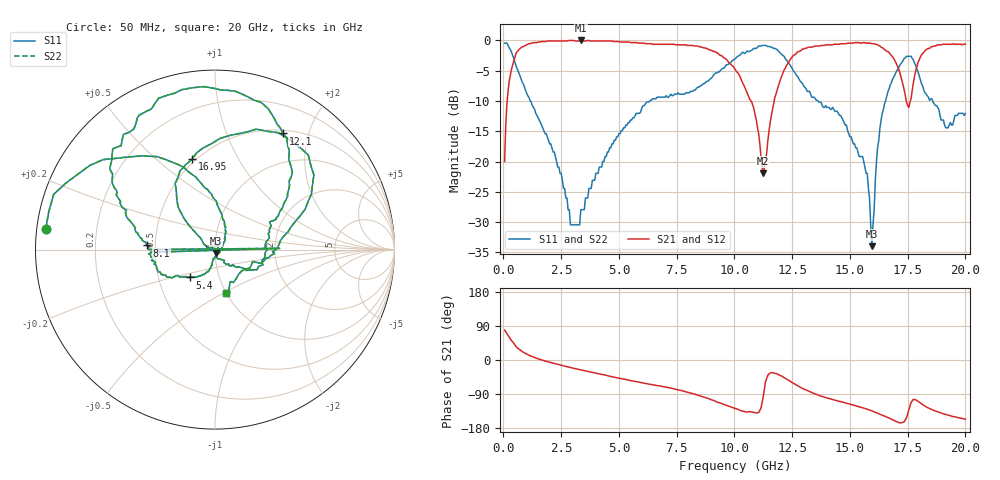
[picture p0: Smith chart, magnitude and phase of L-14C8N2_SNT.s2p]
#	mhz	s	ma	r	50
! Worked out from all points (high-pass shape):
!   400 points, 50 MHz to 20 GHz, reference 50 ohm
!   highest |S21| = 0.00 dB at 3.35 GHz (marker M1); lowest = -21.9 dB at 11.25 GHz (marker M2)
!   |S21| within 3 dB of the highest: 478.4 MHz to 9.61 GHz (9.132 GHz wide, 181 % of centre); 12.44 GHz to 16.9 GHz (4.458 GHz wide, 30.4 % of centre)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
!   lowest |S11| = -34.0 dB at 15.95 GHz (marker M3), VSWR 1.04, Z = 50.7 - j1.9 ohm
!   |S11| at or under -10 dB: 1.169 GHz to 6.331 GHz (5.163 GHz wide, 138 % of centre); 13.62 GHz to 16.54 GHz (2.922 GHz wide, 19.4 % of centre); 18.58 GHz to end of sweep
!   |S22| runs from -34.0 to -0.4 dB; largest |S21 - S12| = 0
!   S11 on the Smith chart (normalised r, x): 50 MHz: 0.03, +0.06; 5.4 GHz: 0.72, -0.23; 8.1 GHz: 0.45, +0.02; 12.1 GHz: 0.54, +1.61; 16.95 GHz: 0.48, +0.66; 20 GHz: 1.00, -0.52
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50  0.95 173.2  0.1 79.0  0.1 79.0  0.95 173.2
550  0.61 121.9  0.79 34.9  0.79 34.9  0.61 121.9
2900  0.03 6.3  1 -19.9  1 -19.9  0.03 6.3
3350  0.04 -81.1  1 -26.3  1 -26.3  0.04 -81.1
3400  0.04 -84.2  1 -26.9  1 -26.9  0.04 -84.2
5400  0.21 -132.3  0.97 -53.0  0.97 -53.0  0.21 -132.3
6700  0.34 -159.0  0.93 -67.8  0.93 -67.8  0.34 -159.0
7750  0.36 -177.6  0.92 -81.3  0.92 -81.3  0.36 -177.6
7800  0.36 1.1  0.92 -82.2  0.92 -82.2  0.36 1.1
7850  0.36 179.9  0.92 -83.0  0.92 -83.0  0.36 179.9
8100  0.38 176.5  0.91 -87.0  0.91 -87.0  0.38 176.5
10050  0.71 143.5  0.57 -128.6  0.57 -128.6  0.71 143.5
11250  0.91 99.3  0.08 -95.9  0.08 -95.9  0.91 99.3
12100  0.75 59.6  0.54 -44.5  0.54 -44.5  0.75 59.6
13350  0.34 26.9  0.88 -86.2  0.88 -86.2  0.34 26.9
15550  0.11 -49.7  0.96 -126.1  0.96 -126.1  0.11 -49.7
15950  0.02 -69.4  0.94 -134.2  0.94 -134.2  0.02 -69.4
16200  0.13 140.1  0.92 -140.5  0.92 -140.5  0.13 140.1
16700  0.4 122.8  0.79 -153.5  0.79 -153.5  0.4 122.8
16950  0.52 104.3  0.68 -161.0  0.68 -161.0  0.52 104.3
17750  0.69 37.0  0.45 -103.8  0.45 -103.8  0.69 37.0
20000  0.25 -75.4  0.93 -156.0  0.93 -156.0  0.25 -75.4
